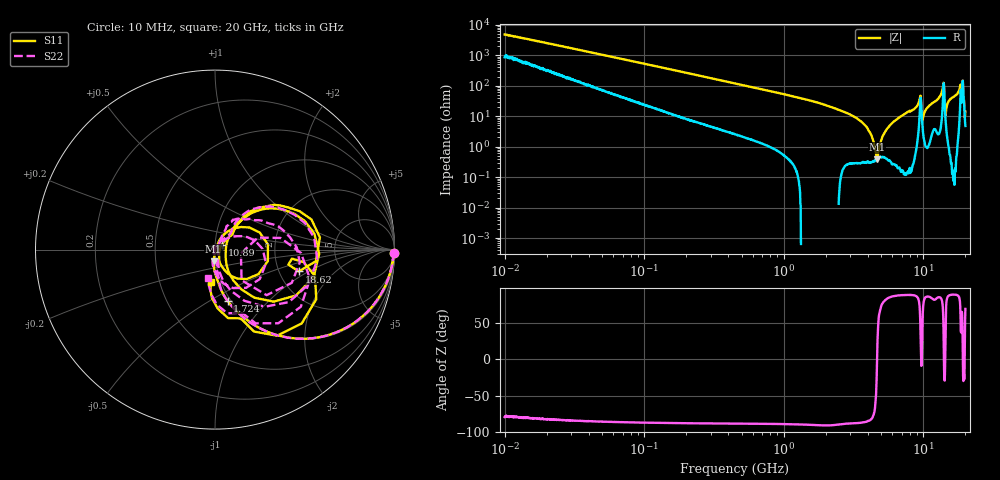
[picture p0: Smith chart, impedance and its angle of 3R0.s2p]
!Keysight Technologies,P5008B,MY61100088,A.16.20.02
!Date: Monday, October 30, 2023 16:35:02
!Correction: S11(C  2-Port  )
!S21(C  2-Port  )
!S12(C  2-Port  )
!S22(C  2-Port  )
!S2P File: Measurements: S11, S21, S12, S22:Log Frequency Sweep
# Hz S  dB  R 50
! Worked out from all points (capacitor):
!   1601 points, 10 MHz to 20 GHz, reference 50 ohm
!   read as one part in series: C = 3.3 pF near 10.39 MHz
!   lowest |Z| = 385 mohm at 4.652 GHz (marker M1)
!   series resonance near 4.659 GHz, so ESL is about 350 pH
!   S11 on the Smith chart (normalised r, x): 10 MHz: 17, -93; 1.724 GHz: 0.97, -0.60; 10.89 GHz: 1.08, +0.05; 18.62 GHz: 2.56, -0.81; 20 GHz: 0.90, -0.33
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1e7  -0.03 -1.2  -33.64 78.5  -33.65 78.5  -0.03 -1.2
3.555162e7  -0.07 -4.0  -23.24 81.2  -23.24 81.2  -0.07 -4.0
1.263918e8  -0.32 -13.5  -12.73 74.2  -12.74 74.2  -0.32 -13.5
4.472136e8  -2.38 -39.9  -3.96 48.9  -3.97 48.9  -2.38 -39.9
1.589917e9  -9.97 -74.3  -0.44 16.3  -0.44 16.3  -9.96 -74.4
1.723645e9  -10.67 -76.2  -0.36 14.6  -0.36 14.6  -10.67 -76.5
4.652055e9  -23.61 -96.9  -0.04 -3.7  -0.04 -3.7  -23.54 -81.7
5.652411e9  -28.32 -95.2  -0.02 -7.4  -0.02 -7.4  -28.15 -83.1
6.999632e9  -36.60 -26.3  0.00 -12.0  -0.00 -12.0  -41.05 -168.3
7.697294e9  -30.67 27.3  -0.00 -14.6  -0.00 -14.6  -31.97 114.9
8.344716e9  -35.12 49.7  -0.00 -17.2  -0.01 -17.2  -34.99 70.7
9.531902e9  -10.57 5.7  -2.80 -24.5  -2.81 -24.6  -10.63 -15.0
9.854205e9  -18.34 -65.6  -0.42 -13.2  -0.42 -13.2  -18.73 -91.9
1.038284e10  -30.23 -41.3  -0.06 -19.3  -0.06 -19.3  -35.49 -111.1
1.088799e10  -26.94 32.7  -0.06 -22.5  -0.07 -22.5  -30.04 60.1
1.141771e10  -21.19 42.5  -0.18 -25.2  -0.18 -25.2  -22.22 51.3
1.361179e10  -7.61 33.1  -1.60 -43.5  -1.60 -43.6  -7.58 34.2
1.44103e10  -16.58 -58.9  -0.66 -14.9  -0.67 -14.9  -17.98 -78.7
1.49685e10  -19.79 41.6  -0.12 -26.9  -0.12 -27.0  -21.05 63.5
1.767617e10  -9.60 44.6  -0.67 -49.7  -0.67 -49.7  -10.28 31.9
1.862442e10  -6.33 -14.6  -4.18 -38.2  -4.19 -38.2  -12.92 -49.1
2e10  -14.93 -96.6  -0.59 -25.9  -0.59 -25.9  -15.89 -103.7
